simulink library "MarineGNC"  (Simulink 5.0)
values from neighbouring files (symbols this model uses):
  D = 6.533    [RRDcontainer.m]    (also in ExObsCtr.m = sqrt(g/L)*T*Dbis*Tinv)
  delta_max = 20    [RRDcontainer.m]
  G = Hmtrx(r_g)' * G_CG * Hmtrx(r_g)    [Gmtrx.m]    (also in ExLQR.m = -K; ExRRD1.m = [ 0 0.0000704  0; ExRRD2.m = [ 0 0.0000704  0)
  M = 1    [ExWindForce.m]    (also in ExRRD1.m = [ 0.01497    0.0003525     -0.0002205; ExRRD2.m = [ 0.01497    0.0003525     -0.0002205; ExObsCtr.m = T*Mbis*Tinv)
  pathlength = pathlength + sqrt( (xpath(j+1)-xpath(j))^2 + (ypath(j+1)-ypath(j))^2)    [order5.m]    (also in order3.m)
  table = table'    [order5.m]    (also in order3.m)
undefined symbols (not defined in the file or in its folder): Acc, feval, K_supply, rate_max, T_supply
libraries: MarineGNC x24, simulink x18
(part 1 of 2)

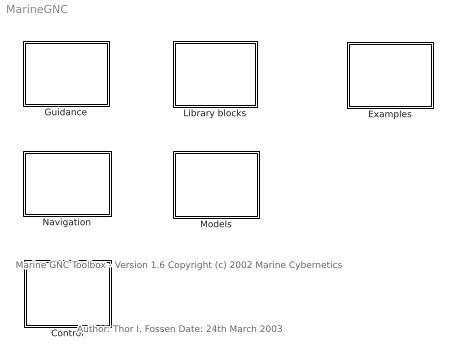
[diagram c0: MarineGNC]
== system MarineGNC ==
  note: Marine GNC Toolbox - Version 1.6 Copyright (c) 2002 Marine Cybernetics
  note: Author: Thor I. Fossen Date: 24th March 2003
  Control : Subsystem
  Examples : Subsystem
  Guidance : Subsystem
  Library blocks : Subsystem
  Models : Subsystem
  Navigation : Subsystem

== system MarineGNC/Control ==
  Ship control systems : Subsystem

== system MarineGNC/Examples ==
  Autopilot wave filter:   compass and yaw gyro : Subsystem
  Autopilot with wave filter: only compass measurement : Subsystem
  "Simulink interface for  m-file vessel models " : Subsystem
  Thruster configuration matrix for supply vessel : Subsystem
  Way-point guidance : Subsystem

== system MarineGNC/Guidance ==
  Reference model : Subsystem  mask(3rd-order reference model){v_max=1.0, zeta_d=1.0, w_d=0.1}
      mask prompts: v_max "Max. velocity:"; zeta_d "Relative damping ratio:"; w_d "Natural frequency:"
      mask help: 3rd-order reference model with velocity saturation.
  Way-point guidance block : Subsystem  mask(Guidance){x_vector=[-800 -500 -200 -50 -200 -250 200 500 500 300 0 -300 -600], y_vector=[100 1800 2000 1500 1000 100 1000 300 -250 -200 100 -600 -1000], method=5th order polynomial, drawmode=off, stop=on, mode=Acc, start=[100 0], final=[0 100], constraint=off}
      mask prompts: x_vector "X value"; y_vector "Y value"; method "Computation method for path generation"; drawmode "Draw an extra plot showing the path with waypoints"; stop "Stop simulation when last waypoint is reached"; mode "Use constraints on acceleration or velocity in the endpoints"; start "Constraints in first waypoint [x, y]. (Only applicable for cubic splines)"; final "Constraints in last waypoint [x, y]. (Only applicable for cubic splines)"; constraint "Use constraints on the derivatives (Only applicable for 5th order)"
      mask help: Way-Point Guidance Block Author: Jørgen Corneliussen Date: 20 November 2002 Creates a three times differentiable path between the waypoints provided. The user can choose between cubic splines and polinomial interpolation. NOTE: You have to supply the actual waypoints for the path generation.
      mask init:
      | if method == 1
      | 	[table, pathlength] = order3(x_vector,y_vector, drawmode, mode, start(1), final(1), start(2), final(2));
      | elseif method == 2
      | 	[table, pathlength] = order5(drawmode, constraint, x_vector, y_vector);
      | else
      | 	disp('Error in block initialization')
      | end

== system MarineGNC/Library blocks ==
  Angle conversion : Subsystem
  Axes transformations : Subsystem
  Equations of motion : Subsystem

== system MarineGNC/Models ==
  Actuators : Subsystem
  Vessels : Subsystem
  "Waves, wind and currents" : Subsystem

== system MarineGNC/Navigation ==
  Wave filters : Subsystem

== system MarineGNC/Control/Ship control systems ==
  Course autopilot : Subsystem  mask(Course Autopilot){T_nomoto=1, K_nomoto=1, Kp=1, Td=0, Ti=0}
      mask prompts: T_nomoto "Nomoto Time Constant: T"; K_nomoto "Nomoto gain: K"; Kp "Proportional Gain: Kp"; Td "Derivative Time: Td"; Ti "Integral Time: Ti"
      mask help: PID Autopilot with reference feedforward.
  DP controller : Subsystem  mask(Nonlinear DP Controller){Kp=diag([1 1 1]), Kd=diag([1 1 1]), Ki=diag([1 1 1])}
      mask prompts: Kp "Proportional Gain Matrix: Kp"; Kd "Derivative Gain Matrix: Kd"; Ki "Integral Gain Matrix: Ki"
      mask help: Nonlinear PID controller for Set-Point Reulation in Surge, Sway and Yaw

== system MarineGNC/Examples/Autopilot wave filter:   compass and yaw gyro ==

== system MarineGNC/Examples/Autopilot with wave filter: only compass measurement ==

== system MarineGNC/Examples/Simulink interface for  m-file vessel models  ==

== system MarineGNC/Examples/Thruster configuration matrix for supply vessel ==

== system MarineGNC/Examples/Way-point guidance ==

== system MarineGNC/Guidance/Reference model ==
  desired position : Inport
  "    " : TransferFcn  Denominator=[1 0]
  "       " : Saturate  UpperLimit=v_max  LowerLimit=-v_max
  "         " : TransferFcn  Denominator=[1 0]
  Sum2 : Sum  Inputs=|+-
  Sum5 : Sum  Inputs=|+-
  damping : Gain  Orientation=left  Gain=2*zeta_d*w_d
  low-pass filter : TransferFcn  Numerator=[w_d^3]  Denominator=[1 w_d]
  spring : Gain  Orientation=left  Gain=w_d*w_d
  "desired position " : Outport  InitialOutput=0
  desired velocity : Outport  Port=2  InitialOutput=0
  desired acceleration : Outport  Port=3  InitialOutput=0
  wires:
  damping/1 -> Sum5/2
  "         "/1 -> "       "/1
  "    "/1 -> "desired position "/1, spring/1
  spring/1 -> Sum2/2
  Sum2/1 -> Sum5/1
  low-pass filter/1 -> Sum2/1
  desired position/1 -> low-pass filter/1
  Sum5/1 -> "         "/1, desired acceleration/1
  "       "/1 -> damping/1, "    "/1, desired velocity/1

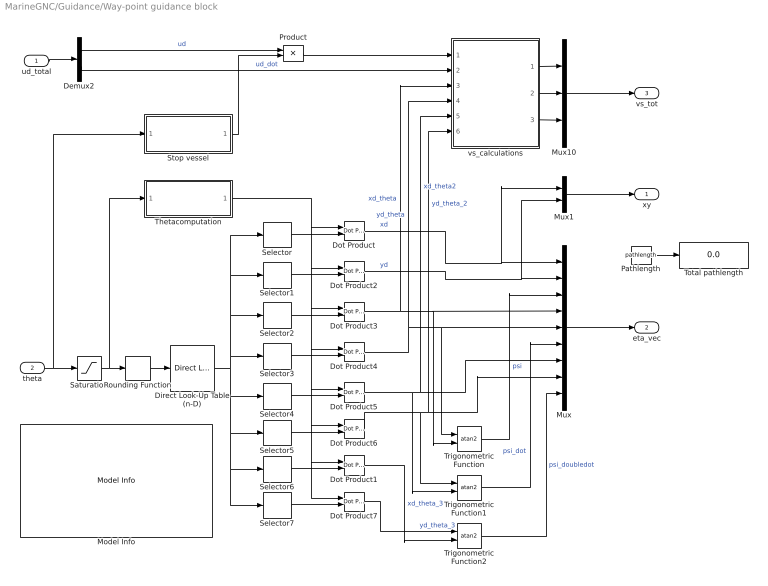
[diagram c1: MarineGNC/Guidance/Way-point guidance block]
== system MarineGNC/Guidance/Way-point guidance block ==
  ud_total : Inport  PortDimensions=2
  theta : Inport  Port=2
  Demux2 : Demux  Outputs=2
  Direct Look-Up Table (n-D) : simulink/Look-Up Tables/Direct Look-Up Table (n-D)  maskTabDims=2  explicitNumDims=1  outDims=Column  tabIsInput=off  mxTable=table  clipFlag=None
  Dot Product{,1..7} (8 alike) : simulink/Math Operations/Dot Product
  Model Info : simulink/Model-Wide Utilities/Model Info  InitialBlockCM=none  BlockCM=None  Frame=on  DisplayStringWithTags=|  HorizontalTextAlignment=Center  LeftAlignmentValue=0.5  SourceBlockDiagram=MarineGNC  TagMaxNumber=20
      | Guidance block.
      | Creates a three times differentiable path 
      | between the provided waypoints. The user 
      | can choose between cubic splines and a 
      | 5th order polynomial.
      | Author: Jørgen Corneliussen
      | Modified: %<ModifiedDate>
      | Version: %<ModelVersion>
  Mux : Mux  Inputs=9
  Mux1 : Mux  Inputs=2
  Mux10 : Mux  Inputs=3
  Pathlength : Constant  Value=pathlength
  Product : Product
  Rounding Function : Rounding
  Saturation : Saturate  UpperLimit=size(table,2) -0.001  LowerLimit=0
  Selector : Selector  Elements=[0*(size(table,1)/8)+1 :1*(size(table,1)/8)]  InputPortWidth=size(table,1)
  Selector1 : Selector  Elements=[1*(size(table,1)/8)+1 :2*(size(table,1)/8)]  InputPortWidth=size(table,1)
  Selector2 : Selector  Elements=[2*(size(table,1)/8)+1 :3*(size(table,1)/8)]  InputPortWidth=size(table,1)
  Selector3 : Selector  Elements=[3*(size(table,1)/8)+1 :4*(size(table,1)/8)]  InputPortWidth=size(table,1)
  Selector4 : Selector  Elements=[4*(size(table,1)/8)+1 :5*(size(table,1)/8)]  InputPortWidth=size(table,1)
  Selector5 : Selector  Elements=[5*(size(table,1)/8)+1 :6*(size(table,1)/8)]  InputPortWidth=size(table,1)
  Selector6 : Selector  Elements=[6*(size(table,1)/8)+1 :7*(size(table,1)/8)]  InputPortWidth=size(table,1)
  Selector7 : Selector  Elements=[7*(size(table,1)/8)+1 :8*(size(table,1)/8)]  InputPortWidth=size(table,1)
  Stop vessel : Subsystem
  Thetacomputation : Subsystem
  Total pathlength : Display
  Trigonometric Function : Trigonometry  Operator=atan2
  Trigonometric Function1 : Trigonometry  Operator=atan2
  Trigonometric Function2 : Trigonometry  Operator=atan2
  vs_calculations : Subsystem
  xy : Outport
  eta_vec : Outport  Port=2
  vs_tot : Outport  Port=3
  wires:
  theta/1 -> Saturation/1, Stop vessel/1(theta)
  ud_total/1 -> Demux2/1
  Thetacomputation/1(thetavector) -> Dot Product/1, Dot Product2/1, Dot Product4/1, Dot Product5/1, Dot Product6/1, Dot Product7/1, Dot Product1/1, Dot Product3/1
  Dot Product/1 -> Mux/1, Mux1/1  "xd"
  Dot Product2/1 -> Mux/2, Mux1/2  "yd"
  Mux/1 -> eta_vec/1
  Dot Product3/1 -> Trigonometric Function/2, Mux/4, vs_calculations/3(xd_theta)  "xd_theta"
  Dot Product4/1 -> Mux/5, Trigonometric Function/1, vs_calculations/4(yd_theta)  "yd_theta"
  Dot Product5/1 -> Trigonometric Function1/2, Mux/7, vs_calculations/5(xd_theta_2)  "xd_theta2"
  Dot Product6/1 -> Trigonometric Function1/1, Mux/8, vs_calculations/6(yd_theta_2)  "yd_theta_2"
  Dot Product1/1 -> Trigonometric Function2/2  "xd_theta_3"
  Dot Product7/1 -> Trigonometric Function2/1  "yd_theta_3"
  Trigonometric Function/1 -> Mux/3  "psi"
  Trigonometric Function1/1 -> Mux/6  "psi_dot"
  Trigonometric Function2/1 -> Mux/9  "psi_doubledot"
  Mux10/1 -> vs_tot/1
  vs_calculations/1(vs) -> Mux10/1
  vs_calculations/3(vs_t) -> Mux10/3
  vs_calculations/2(vs_theta) -> Mux10/2
  Saturation/1 -> Rounding Function/1, Thetacomputation/1(theta)
  Selector/1 -> Dot Product/2
  Selector1/1 -> Dot Product2/2
  Selector2/1 -> Dot Product3/2
  Selector3/1 -> Dot Product4/2
  Selector4/1 -> Dot Product5/2
  Selector5/1 -> Dot Product6/2
  Selector6/1 -> Dot Product1/2
  Selector7/1 -> Dot Product7/2
  Direct Look-Up Table (n-D)/1 -> Selector/1, Selector1/1, Selector2/1, Selector3/1, Selector4/1, Selector5/1, Selector7/1, Selector6/1
  Rounding Function/1 -> Direct Look-Up Table (n-D)/1
  Demux2/1 -> Product/1  "ud"
  Product/1 -> vs_calculations/1(ud)
  Stop vessel/1(stopsignal) -> Product/2
  Demux2/2 -> vs_calculations/2(ud_dot)  "ud_dot"
  Mux1/1 -> xy/1
  Pathlength/1 -> Total pathlength/1

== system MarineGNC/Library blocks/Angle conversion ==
  deg to [-180 180] : Subsystem
  rad to [-pi pi] : Subsystem

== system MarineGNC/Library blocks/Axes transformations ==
  6 DOF transformation : Subsystem
  Euler angles to rotation matrix : Subsystem
  Euler angles to attitude transformation matrix : Subsystem
  "Rotataion matrix in yaw " : Subsystem
  Transformation of generalized force : Subsystem
  Transposed rotation  matrix in yaw : Subsystem

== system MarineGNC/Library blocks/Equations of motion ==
  3 DOF Eqs. of motion : Subsystem
  3 to 6 DOF : Subsystem
  6 DOF Eqs. of motion : Subsystem
  6 to 3 DOF : Selector  Elements=[1 2 6]  InputPortWidth=6

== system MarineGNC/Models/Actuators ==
  note: Propellers
  note: Thruster configuration blocks
  note: Machines
  Column vector t1 : Subsystem
  Propeller : Subsystem  mask(Propeller){rpm_max=5*(180/pi)}
      mask prompts: rpm_max "Max RPM:"
  Steering machine : Subsystem
  T(alpha) : Subsystem

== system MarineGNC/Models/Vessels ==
  note: Nomoto models (1 DOF)
  note: Low-Speed Models (3 DOF)
  note: Low-Speed Models (6 DOF) 6 DOF interface for 3 DOF models
  note: Interface to m-file models
  3 to 6 DOF : MarineGNC/Library blocks/Equations of motion/3 to 6 DOF
  3 to 6 DOF1 : MarineGNC/Library blocks/Equations of motion/3 to 6 DOF
  6 to 3 DOF : Selector  Elements=[1 2 6]  InputPortWidth=6
  CyberShipII : Subsystem  LoadFcn=initCS2
  Mariner class cargo ship  (2nd -order) : Subsystem  mask(Container ship (2nd-order model)){rate_max=5*(pi/180), delta_max=20*(pi/180), K=0.185, T1=118, T2=7.8, T3=18.5}
      mask prompts: rate_max "Max rudder rate: rate_max (rad/s)"; delta_max "Max rudder angle: delta_max (rad)"; K "Gain constant: K (1/s)"; T1 "Time constant: T1 (s)"; T2 "Time constant: T2 (s)"; T3 "Time constant: T3 (s)"
  Semi-sub : Subsystem  InitFcn=load MDGmodels/rig  mask(Semi-submersiblel (6 DOF)){D=D, G=G, M=M}
      mask prompts: D "Linear damping matrix: D"; G "Spring matrix G:"; M "System inertia matrix: M"
      mask help: Semi-submersible low-speed model for DP. Inputs: tau = 6 DOF control input vector (generalized force) Outputs: eta = [x, y, z, phi, theta, psi]' nu = [u, v, w, p, q, r]'
  Supply vessel : Subsystem  mask(Supply Vessel (surge, sway and yaw)){D=[5.0242e4 0 0; 0 2.7229e5 -4.3933e6; 0 -4.3933e6 4.1894e8], Minv=inv( [5.3122e6 0 0; 0 8.2831e6 0; 0 0 3.7454e9] )}
      mask prompts: D "Linear damping matrix: D"; Minv "Inverse inertia matrix: Minv"
      mask help: DP model Inputs: tau = 3 DOF control input vector (generalized force) Outputs: eta = [x, y, psi]' nu = [u, v, r]'
  Supply vessel1 : MarineGNC/Models/Vessels/Supply vessel  D=[5.0242e4 0 0; 0 2.7229e5 -4.3933e6; 0 -4.3933e6 4.1894e8]  Minv=inv( [5.3122e6 0 0; 0 8.2831e6 0; 0 0 3.7454e9] )
  Tanker (1st-order) : Subsystem  mask(Tanker (Nomoto 1st.-order)){rate_max=5*(pi/180), delta_max=20*(pi/180), K=-0.019, T=-153.7}
      mask prompts: rate_max "Max rudder rate: rate_max (rad/s):"; delta_max "Max rudder angle: delta_max  (rad)"; K "Gain constant: K (1/s)"; T "Time constant: T (s)"
      mask help: Tanker: Nomoto 1st-order model Input: delta_c = rudder angle command (rad) Outputs: psi = yaw angle (rad) r = yaw rate (rad) delta = rudder angle from steering machine (rad)
  Tanker (2nd-order) : Subsystem  mask(Tanker (Nomoto 2nd-order model)){rate_max=5*(pi/180), delta_max=20*(pi/180), K=-0.019, T1=-124.1, T2=16.4, T3=46}
      mask prompts: rate_max "Max rudder rate: rate_max (rad/s)"; delta_max "Max rudder angle: delta_max (rad)"; K "Gain constant: K (1/s)"; T1 "Time constant: T1 (s)"; T2 "Time constant: T2 (s)"; T3 "Time constant: T3 (s)"
      mask help: Tanker: Nomoto 2nd-order model Input: delta_c = rudder angle command (rad) Outputs: psi = yaw angle (rad) r = yaw rate (rad) delta = rudder angle from steering machine (rad)
  m-file interface : Subsystem  mask(m-file vessel model interface){vessmodel=, dimu_model=, dimx_model=}
      mask prompts: vessmodel "m-file vessel model"; dimu_model "dim u"; dimx_model "dim x"
      mask help: Simulink interface to the GNC toolbox m-file vessel models, type: >help vesselmodels in the Matlab command window. A Simulink demo file is found under examples (demomf.mdl). Inputs/outputs: u = control input vector of dimension dimu xo = initial state vector of dimension dimx x = state vector of dimension dimu
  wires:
  Supply vessel1/1 -> 3 to 6 DOF/1
  Supply vessel1/2 -> 3 to 6 DOF1/1
  6 to 3 DOF/1 -> Supply vessel1/1

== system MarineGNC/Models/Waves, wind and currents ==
  Linear 2nd-order  wave spectrum : Subsystem  mask{sigma=1, w_0=1, lambda=0.1}
      mask prompts: sigma "Wave spectrum gain: sigma  (m)"; w_0 "Wave spectrum peak frequency: w_0  (rad/s)"; lambda "Rrelative damping ratio: lambda"
      mask init:
      | w = 0.01:0.1:3*w_0;

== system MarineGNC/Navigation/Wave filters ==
  Passive autopilot wave filter 1 : Subsystem  mask(wave spectrum damping ratio){lambda=0.1, w_o=1.2, K4=0.1, K5=0.01, w_c=1.3, T=100, K=1, T_b=100}
      mask prompts: lambda "Relative damping ratio of wave spectrum: lambda"; w_o "Peak frequency of wave spectrum: w_o (rad/s)"; K4 "Yaw rate observer gain: K4"; K5 "Bias observer gain: K5"; w_c "Filter cut-off frequency: w_c (rad/s)"; T "Nomoto time constant: T (s)"; K "Nomoto gain: K (1/s)"; T_b "Rudder bias time constant: T_b (s)"
  Passive autopilot wave filter 2 : Subsystem  mask(wave spectrum damping ratio){lambda=0.1, w_o=1.2, K4=0.1, zeta_n=0.01, w_c=2, T_b=100}
      mask prompts: lambda "Relative damping ratio of wave spectrum: lambda"; w_o "Peak frequency of wave spectrum: w_o (rad/s)"; K4 "Bias observer gain: K4"; zeta_n "Relative damping ratio in gyro notch filter: zeta_n"; w_c "Filter cut-off frequency: w_c (rad/s)"; T_b "Bias time constant: T_b (s)"

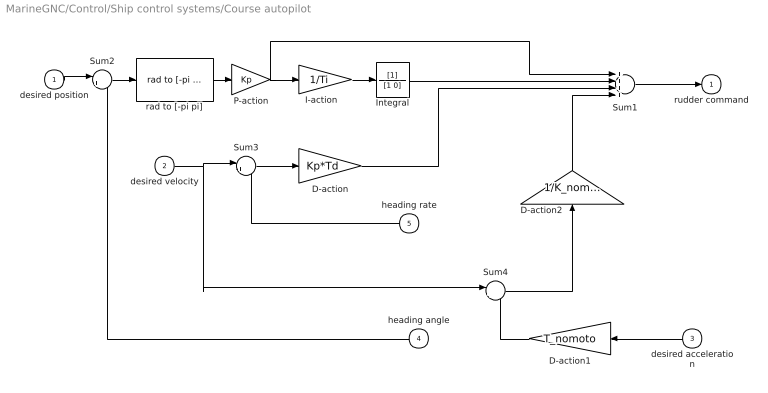
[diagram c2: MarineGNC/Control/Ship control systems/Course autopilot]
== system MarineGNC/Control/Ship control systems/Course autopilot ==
  desired position : Inport
  desired velocity : Inport  Port=2
  desired acceleration : Inport  Orientation=left  Port=3
  heading angle : Inport  Orientation=left  Port=4
  heading rate : Inport  Orientation=left  Port=5
  D-action : Gain  Gain=Kp*Td
  D-action1 : Gain  Orientation=left  Gain=T_nomoto
  D-action2 : Gain  Orientation=up  Gain=1/K_nomoto
  "I-action   " : Gain  Gain=1/Ti
  Integral : TransferFcn  Denominator=[1 0]
  P-action : Gain  Gain=Kp
  Sum1 : Sum  Inputs=++++
  Sum2 : Sum  Inputs=|+-
  Sum3 : Sum  Inputs=|+-
  Sum4 : Sum  Inputs=|++
  rad to [-pi pi] : MarineGNC/Library blocks/Angle conversion/rad to [-pi pi]  SimViewingDevice=off  DataTypeOverride=UseLocalSettings  MinMaxOverflowLogging=UseLocalSettings
  rudder command : Outport  InitialOutput=0
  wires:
  P-action/1 -> Sum1/1, "I-action   "/1
  "I-action   "/1 -> Integral/1
  D-action/1 -> Sum1/3
  Sum1/1 -> rudder command/1
  Integral/1 -> Sum1/2
  Sum3/1 -> D-action/1
  heading angle/1 -> Sum2/2
  desired acceleration/1 -> D-action1/1
  heading rate/1 -> Sum3/2
  desired velocity/1 -> Sum3/1, Sum4/1
  D-action1/1 -> Sum4/2
  Sum4/1 -> D-action2/1
  D-action2/1 -> Sum1/4
  Sum2/1 -> rad to [-pi pi]/1
  rad to [-pi pi]/1 -> P-action/1
  desired position/1 -> Sum2/1

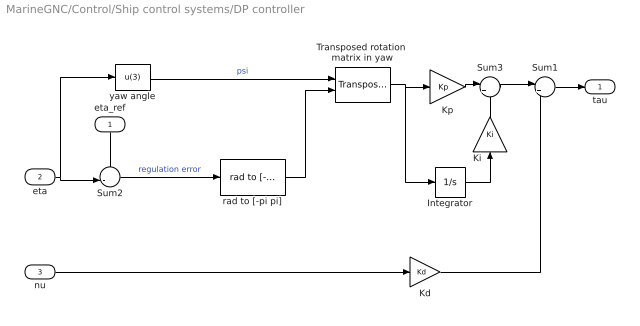
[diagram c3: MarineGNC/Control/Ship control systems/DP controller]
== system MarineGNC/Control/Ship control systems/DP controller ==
  eta_ref : Inport  Orientation=down
  eta : Inport  Port=2
  nu : Inport  Port=3
  Integrator : Integrator
  Kd : Gain  Gain=Kd  Multiplication=Matrix(K*u)
  Ki : Gain  Orientation=up  Gain=Ki  Multiplication=Matrix(K*u)
  Kp : Gain  Gain=Kp  Multiplication=Matrix(K*u)
  Sum1 : Sum  Inputs=|+-
  Sum2 : Sum  Inputs=+-|
  Sum3 : Sum  Inputs=|++
  Transposed rotation  matrix in yaw : MarineGNC/Library blocks/Axes transformations/Transposed rotation  matrix in yaw
  rad to [-pi pi] : MarineGNC/Library blocks/Angle conversion/rad to [-pi pi]  SimViewingDevice=off  DataTypeOverride=UseLocalSettings  MinMaxOverflowLogging=UseLocalSettings
  yaw angle : Fcn  Expr=u(3)
  tau : Outport  InitialOutput=0
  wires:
  Transposed rotation  matrix in yaw/1 -> Integrator/1, Kp/1
  Ki/1 -> Sum3/2
  Sum3/1 -> Sum1/1
  Kp/1 -> Sum3/1
  Integrator/1 -> Ki/1
  Kd/1 -> Sum1/2
  nu/1 -> Kd/1
  yaw angle/1 -> Transposed rotation  matrix in yaw/1  "psi"
  eta/1 -> yaw angle/1, Sum2/2
  Sum1/1 -> tau/1
  eta_ref/1 -> Sum2/1
  Sum2/1 -> rad to [-pi pi]/1  "regulation error"
  rad to [-pi pi]/1 -> Transposed rotation  matrix in yaw/2

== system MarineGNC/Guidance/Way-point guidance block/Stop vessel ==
  theta : Inport
  If endpoint1 : If  IfExpression=u1 > size(table,2)
  Merge : Merge
  Model Info : simulink/Model-Wide Utilities/Model Info  InitialBlockCM=None  BlockCM=None  Frame=on  DisplayStringWithTags=|  HorizontalTextAlignment=Center  LeftAlignmentValue=0.5  SourceBlockDiagram=demowpt  TagMaxNumber=20
      | Stop vessel
      | 
      | This subsystem performs an action when
      | the vessel reaches the last waypoint. The 
      | simultation is either stopped, or the desired 
      | speed is set to zero.
      | 
      | Author: Jørgen Corneliussen
      | Modified: %<ModifiedDate>
      | Version: %<ModelVersion>
  Reached endpoint : Subsystem  TreatAsAtomicUnit=on
  Still travelling : Subsystem  TreatAsAtomicUnit=on
  stopsignal : Outport
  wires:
  Still travelling/1(one) -> Merge/2
  theta/1 -> If endpoint1/1
  If endpoint1/1 -> Reached endpoint/Action
  Reached endpoint/1(zero) -> Merge/1
  Merge/1 -> stopsignal/1
  If endpoint1/2 -> Still travelling/Action

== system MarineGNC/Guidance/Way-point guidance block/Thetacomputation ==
  theta : Inport
  5th order algorithm : Subsystem  TreatAsAtomicUnit=on
  Constant1 : Constant  Value=method
  Cubic splines : Subsystem  TreatAsAtomicUnit=on
  If endpoint1 : If  IfExpression=u1 == 1
  Model Info : simulink/Model-Wide Utilities/Model Info  InitialBlockCM=None  BlockCM=None  Frame=on  DisplayStringWithTags=|  HorizontalTextAlignment=Center  LeftAlignmentValue=0.5  SourceBlockDiagram=demowpt  TagMaxNumber=20
      | Thetacomputation
      | This subsystem returns a vector containing 
      | different orders of theta.
      | 
      | If cubic splines is used, the system returns:
      | [th^3 th^2 th 1]
      | 
      | If the 5th order polynomial is used, it returns:
      | [th^5 th^4 th^3 th^2 th 1]
      | 
      | Author: Jørgen Corneliussen
      | Modified: %<ModifiedDate>
      | Version: %<ModelVersion>
  Multiport Switch : MultiPortSwitch  Inputs=2
  Selector : Selector  Elements=[1:size(table,1)/8]  InputPortWidth=6
  thetavector : Outport
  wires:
  If endpoint1/1 -> Cubic splines/Action  "cubic"
  If endpoint1/2 -> 5th order algorithm/Action
  Constant1/1 -> If endpoint1/1, Multiport Switch/1
  theta/1 -> 5th order algorithm/1(theta), Cubic splines/1(theta)
  5th order algorithm/1(theta_vector) -> Multiport Switch/3
  Selector/1 -> thetavector/1
  Cubic splines/1(theta_vector) -> Multiport Switch/2
  Multiport Switch/1 -> Selector/1

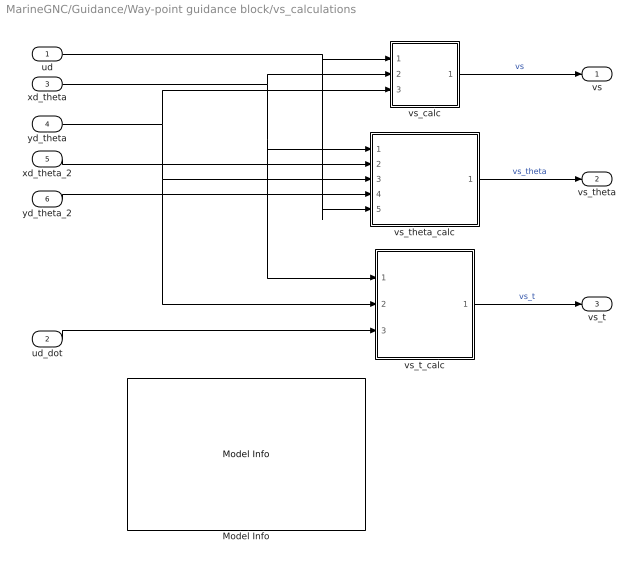
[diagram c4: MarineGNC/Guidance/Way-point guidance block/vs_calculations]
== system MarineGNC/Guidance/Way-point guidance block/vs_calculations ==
  ud : Inport
  ud_dot : Inport  Port=2
  xd_theta : Inport  Port=3
  yd_theta : Inport  Port=4
  xd_theta_2 : Inport  Port=5
  yd_theta_2 : Inport  Port=6
  Model Info : simulink/Model-Wide Utilities/Model Info  InitialBlockCM=None  BlockCM=None  Frame=on  DisplayStringWithTags=|  HorizontalTextAlignment=Center  LeftAlignmentValue=0.5  SourceBlockDiagram=demowpt  TagMaxNumber=20
      | vs_calculations
      | 
      | This subsystem returns a vector containing 
      | the  speed assignment along the path.
      | The vector contains the desired speed, and 
      | the derivative of the desired speed with regards
      |  to theta and with regards to time.
      | 
      | Author: Jørgen Corneliussen
      | Modified: %<ModifiedDate>
      | Version: %<ModelVersion>
  vs_calc : Subsystem
  vs_t_calc : Subsystem
  vs_theta_calc : Subsystem
  vs : Outport
  vs_theta : Outport  Port=2
  vs_t : Outport  Port=3
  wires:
  vs_calc/1(vs) -> vs/1  "vs"
  vs_theta_calc/1(vs_theta) -> vs_theta/1  "vs_theta"
  vs_t_calc/1(vs_t) -> vs_t/1  "vs_t"
  ud/1 -> vs_calc/1(ud), vs_theta_calc/5(ud)
  ud_dot/1 -> vs_t_calc/3(ud_dot)
  xd_theta/1 -> vs_calc/2(xd_theta), vs_theta_calc/1(xd_theta), vs_t_calc/1(xd_theta)
  yd_theta/1 -> vs_calc/3(yd_theta), vs_theta_calc/3(yd_theta), vs_t_calc/2(yd_theta)
  xd_theta_2/1 -> vs_theta_calc/2(xd_theta_2)
  yd_theta_2/1 -> vs_theta_calc/4(yd_theta_2)

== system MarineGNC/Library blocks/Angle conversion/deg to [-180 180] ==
  y (deg) : Inport
  Constant : Constant  Value=180
  Constant1 : Constant  Value=-180
  Data Type Conversion : DataTypeConversion  DataType=double
  "Data Type Conversion  " : DataTypeConversion  DataType=double
  Relational Operator : RelationalOperator  Operator=>
  Relational Operator1 : RelationalOperator  Operator=<
  Sum2 : Sum  Inputs=+++
  twopi : Gain  Gain=-2*180
  "twopi  " : Gain  Gain=2*180
  -180<y180 : Outport  InitialOutput=0
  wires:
  Constant/1 -> Relational Operator/2
  Relational Operator/1 -> Data Type Conversion/1
  Constant1/1 -> Relational Operator1/2
  Relational Operator1/1 -> "Data Type Conversion  "/1
  twopi/1 -> Sum2/1
  "twopi  "/1 -> Sum2/3
  Sum2/1 -> -180<y180/1  "add"
  y (deg)/1 -> Sum2/2, Relational Operator1/1, Relational Operator/1
  Data Type Conversion/1 -> twopi/1
  "Data Type Conversion  "/1 -> "twopi  "/1

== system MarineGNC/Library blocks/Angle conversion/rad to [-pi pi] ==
  y (rad) : Inport
  Constant : Constant  Value=pi
  "Constant " : Constant  Value=-pi
  Data Type Conversion : DataTypeConversion  DataType=double
  Data Type Conversion1 : DataTypeConversion  DataType=double
  Relational Operator : RelationalOperator  Operator=>
  Relational Operator1 : RelationalOperator  Operator=<
  Sum2 : Sum  Inputs=+++
  two pi : Gain  Gain=-2*pi
  "two pi  " : Gain  Gain=2*pi
  -pi<y<pi : Outport  InitialOutput=0
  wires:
  Constant/1 -> Relational Operator/2
  Relational Operator/1 -> Data Type Conversion/1
  "Constant "/1 -> Relational Operator1/2
  Relational Operator1/1 -> Data Type Conversion1/1
  two pi/1 -> Sum2/1
  "two pi  "/1 -> Sum2/3
  Sum2/1 -> -pi<y<pi/1  "add"
  y (rad)/1 -> Sum2/2, Relational Operator1/1, Relational Operator/1
  Data Type Conversion/1 -> two pi/1
  Data Type Conversion1/1 -> "two pi  "/1

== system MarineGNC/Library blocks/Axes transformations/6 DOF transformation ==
  note: Theta
  note: v
  note: omega
  eta : Inport
  nu : Inport  Port=2
  Euler angles to rotation matrix : MarineGNC/Library blocks/Axes transformations/Euler angles to rotation matrix
  Euler angles to attitude transformation matrix : MarineGNC/Library blocks/Axes transformations/Euler angles to attitude transformation matrix
  Mux : Mux  Inputs=2
  Product : Product  Inputs=**  Multiplication=Matrix(*)  ShowAdditionalParam=on
  Product1 : Product  Inputs=**  Multiplication=Matrix(*)  ShowAdditionalParam=on
  Selector : Selector  Elements=[4 5 6]  InputPortWidth=6
  Selector1 : Selector  Elements=[1 2 3]  InputPortWidth=6
  Selector2 : Selector  Elements=[4 5 6]  InputPortWidth=6
  J(eta)*nu : Outport
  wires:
  Selector/1 -> Euler angles to rotation matrix/1, Euler angles to attitude transformation matrix/1
  eta/1 -> Selector/1
  Euler angles to rotation matrix/1 -> Product/1
  nu/1 -> Selector1/1, Selector2/1
  Selector1/1 -> Product/2
  Selector2/1 -> Product1/2
  Euler angles to attitude transformation matrix/1 -> Product1/1
  Product/1 -> Mux/1
  Mux/1 -> J(eta)*nu/1
  Product1/1 -> Mux/2

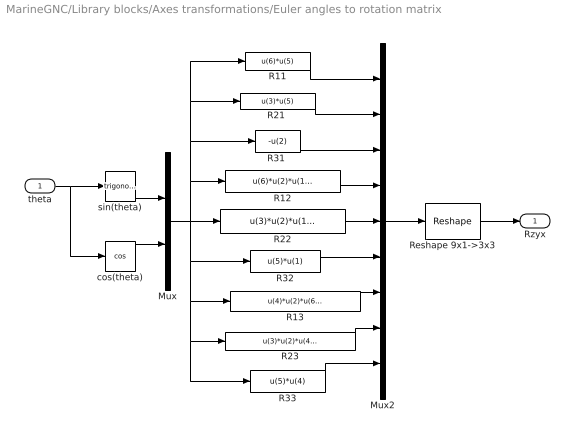
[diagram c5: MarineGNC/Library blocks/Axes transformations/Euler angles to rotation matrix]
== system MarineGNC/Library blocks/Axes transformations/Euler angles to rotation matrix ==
  theta : Inport
  Mux : Mux  Inputs=2
  Mux2 : Mux  Inputs=9
  R11 : Fcn  Expr=u(6)*u(5)
  R12 : Fcn  Expr=u(6)*u(2)*u(1)-u(3)*u(4)
  R13 : Fcn  Expr=u(4)*u(2)*u(6)+u(3)*u(1)
  "R21 " : Fcn  Expr=u(3)*u(5)
  R22 : Fcn  Expr=u(3)*u(2)*u(1)+u(6)*u(4)
  R23 : Fcn  Expr=u(3)*u(2)*u(4)-u(6)*u(1)
  "R31 " : Fcn  Expr=-u(2)
  R32 : Fcn  Expr=u(5)*u(1)
  R33 : Fcn  Expr=u(5)*u(4)
  Reshape 9x1->3x3 : simulink/Math Operations/Reshape  OutputDimensionality=Customize  OutputDimensions=[3,3]
  cos(theta) : Trigonometry  Operator=cos
  sin(theta) : Trigonometry
  Rzyx : Outport  InitialOutput=0
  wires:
  R11/1 -> Mux2/1
  Mux2/1 -> Reshape 9x1->3x3/1
  Reshape 9x1->3x3/1 -> Rzyx/1
  sin(theta)/1 -> Mux/1
  cos(theta)/1 -> Mux/2
  theta/1 -> sin(theta)/1, cos(theta)/1
  Mux/1 -> R32/1, R13/1, R33/1, R23/1, R22/1, "R31 "/1, R11/1, "R21 "/1, R12/1
  R23/1 -> Mux2/8
  R13/1 -> Mux2/7
  R22/1 -> Mux2/5
  R12/1 -> Mux2/4
  "R31 "/1 -> Mux2/3
  "R21 "/1 -> Mux2/2
  R32/1 -> Mux2/6
  R33/1 -> Mux2/9

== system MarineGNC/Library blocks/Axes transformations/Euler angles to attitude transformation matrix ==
  theta : Inport
  Constant : Constant
  "Constant " : Constant  Value=0
  Mux2 : Mux  Inputs=9
  Reshape 9x1->3x3 : simulink/Math Operations/Reshape  OutputDimensionality=Customize  OutputDimensions=[3,3]
  "T21 " : Fcn  Expr=sin(u(1))*tan(u(2))
  T22 : Fcn  Expr=cos(u(1))
  T23 : Fcn  Expr=sin(u(1))/cos(u(2))
  "T31 " : Fcn  Expr=cos(u(1))*tan(u(2))
  T32 : Fcn  Expr=-sin(u(1))
  T33 : Fcn  Expr=cos(u(1))/cos(u(2))
  T : Outport  InitialOutput=0
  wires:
  Constant/1 -> Mux2/1
  Mux2/1 -> Reshape 9x1->3x3/1
  Reshape 9x1->3x3/1 -> T/1
  theta/1 -> T23/1, T33/1, T32/1, "T31 "/1, T22/1, "T21 "/1
  T23/1 -> Mux2/6
  T22/1 -> Mux2/5
  T33/1 -> Mux2/9
  "Constant "/1 -> Mux2/2, Mux2/3
  "T21 "/1 -> Mux2/4
  "T31 "/1 -> Mux2/7
  T32/1 -> Mux2/8

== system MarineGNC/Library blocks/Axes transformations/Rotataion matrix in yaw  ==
  psi : Inport
  nu : Inport  Port=2
  Fcn : Fcn  Expr=cos(u(1))*u(2)-sin(u(1))*u(3)
  Fcn1 : Fcn  Expr=sin(u(1))*u(2)+cos(u(1))*u(3)
  Fcn2 : Fcn  Expr=u(4)
  Mux : Mux  Inputs=2
  Mux1 : Mux  Inputs=3
  R*nu : Outport
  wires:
  Mux/1 -> Fcn2/1, Fcn1/1, Fcn/1
  Fcn/1 -> Mux1/1  "x_dot"
  Fcn1/1 -> Mux1/2  "y_dot"
  Fcn2/1 -> Mux1/3  "psi_dot"
  Mux1/1 -> R*nu/1  "eta_dot"
  psi/1 -> Mux/1
  nu/1 -> Mux/2

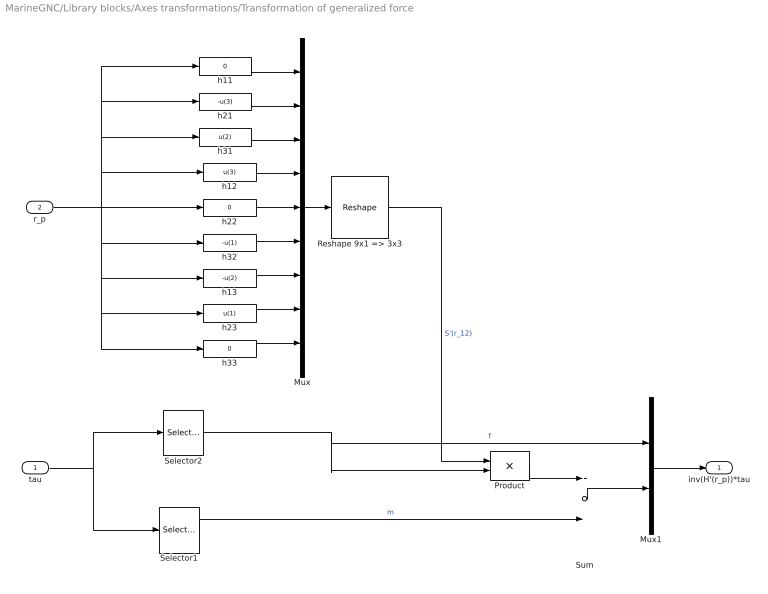
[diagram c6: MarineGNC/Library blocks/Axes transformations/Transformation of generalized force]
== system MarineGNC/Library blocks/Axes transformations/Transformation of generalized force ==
  tau : Inport
  r_p : Inport  Port=2
  Mux : Mux  Inputs=9
  Mux1 : Mux  Inputs=2
  Product : Product  Multiplication=Matrix(*)
  Reshape 9x1 => 3x3 : simulink/Math Operations/Reshape  OutputDimensionality=Customize  OutputDimensions=[3,3]
  Selector1 : Selector  Elements=[4 5 6]  InputPortWidth=6
  Selector2 : Selector  Elements=[1 2 3]  InputPortWidth=6
  Sum : Sum
  h11 : Fcn  Expr=0
  h12 : Fcn  Expr=u(3)
  h13 : Fcn  Expr=-u(2)
  h21 : Fcn  Expr=-u(3)
  h22 : Fcn  Expr=0
  h23 : Fcn  Expr=u(1)
  h31 : Fcn  Expr=u(2)
  h32 : Fcn  Expr=-u(1)
  h33 : Fcn  Expr=0
  inv(H'(r_p))*tau : Outport
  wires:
  tau/1 -> Selector1/1, Selector2/1
  Selector1/1 -> Sum/2  "m"
  Mux/1 -> Reshape 9x1 => 3x3/1
  Reshape 9x1 => 3x3/1 -> Product/1  "S'(r_12)"
  h11/1 -> Mux/1
  h21/1 -> Mux/2
  h31/1 -> Mux/3
  h12/1 -> Mux/4
  h22/1 -> Mux/5
  h32/1 -> Mux/6
  h13/1 -> Mux/7
  h23/1 -> Mux/8
  h33/1 -> Mux/9
  r_p/1 -> h11/1, h21/1, h31/1, h12/1, h22/1, h32/1, h13/1, h23/1, h33/1
  Mux1/1 -> inv(H'(r_p))*tau/1
  Selector2/1 -> Mux1/1, Product/2  "f"
  Sum/1 -> Mux1/2
  Product/1 -> Sum/1

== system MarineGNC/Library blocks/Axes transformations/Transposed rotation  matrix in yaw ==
  psi : Inport
  nu : Inport  Port=2
  Mux : Mux  Inputs=2
  Mux1 : Mux  Inputs=3
  Row1 : Fcn  Expr=cos(u(1))*u(2)+sin(u(1))*u(3)
  Row2 : Fcn  Expr=-sin(u(1))*u(2)+cos(u(1))*u(3)
  Row3 : Fcn  Expr=u(4)
  Out1 : Outport
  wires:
  nu/1 -> Mux/2
  psi/1 -> Mux/1
  Mux1/1 -> Out1/1
  Row3/1 -> Mux1/3
  Row2/1 -> Mux1/2
  Row1/1 -> Mux1/1
  Mux/1 -> Row1/1, Row2/1, Row3/1

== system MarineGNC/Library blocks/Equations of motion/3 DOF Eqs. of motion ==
  M : Inport
  tau : Inport  Port=2
  Integrator1 : Integrator
  Integrator2 : Integrator
  Product : Product  Inputs=/*  Multiplication=Matrix(*)
  "Rotataion matrix in yaw " : MarineGNC/Library blocks/Axes transformations/Rotataion matrix in yaw 
  Selector2 : Selector  Elements=[3]  InputPortWidth=3
  eta : Outport
  nu : Outport  Port=2
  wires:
  M/1 -> Product/1
  tau/1 -> Product/2
  Product/1 -> Integrator1/1  "d(nu)/dt"
  Integrator1/1 -> "Rotataion matrix in yaw "/2, nu/1  "nu"
  "Rotataion matrix in yaw "/1 -> Integrator2/1  "d(eta)/dt"
  Integrator2/1 -> Selector2/1, eta/1  "eta"
  Selector2/1 -> "Rotataion matrix in yaw "/1  "psi"

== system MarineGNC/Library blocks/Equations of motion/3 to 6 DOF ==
  In1 : Inport
  Constant : Constant  Value=0
  Mux1 : Mux  Inputs=2
  Selector : Selector  Elements="[1 2  4 4 4 3]"  InputPortWidth=4
  Out1 : Outport
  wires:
  Selector/1 -> Out1/1
  In1/1 -> Mux1/1
  Constant/1 -> Mux1/2
  Mux1/1 -> Selector/1

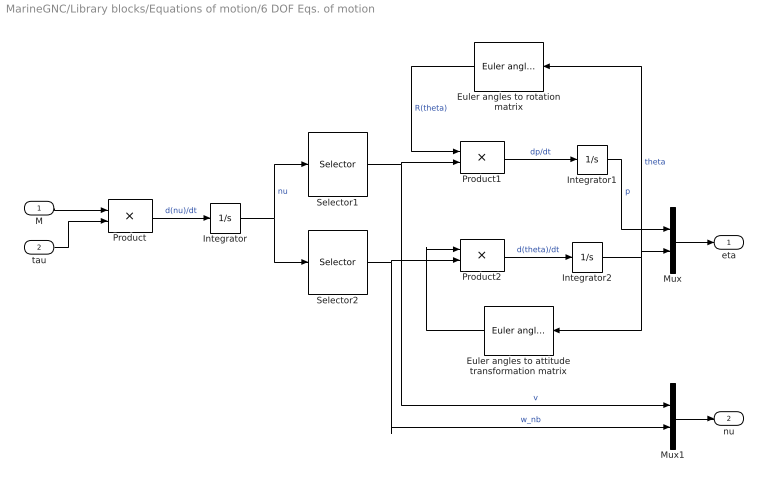
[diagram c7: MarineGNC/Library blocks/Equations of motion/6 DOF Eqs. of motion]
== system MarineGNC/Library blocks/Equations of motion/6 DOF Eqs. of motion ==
  M : Inport
  tau : Inport  Port=2
  Euler angles to rotation matrix : MarineGNC/Library blocks/Axes transformations/Euler angles to rotation matrix  Orientation=left
  Euler angles to attitude transformation matrix : MarineGNC/Library blocks/Axes transformations/Euler angles to attitude transformation matrix  Orientation=left
  Integrator : Integrator
  Integrator1 : Integrator
  Integrator2 : Integrator
  Mux : Mux  Inputs=2
  Mux1 : Mux  Inputs=2
  Product : Product  Inputs=/*  Multiplication=Matrix(*)
  Product1 : Product  Inputs=**  Multiplication=Matrix(*)
  Product2 : Product  Inputs=**  Multiplication=Matrix(*)
  Selector1 : Selector  Elements=[1 2 3]  InputPortWidth=6
  Selector2 : Selector  Elements=[4 5 6]  InputPortWidth=6
  eta : Outport
  nu : Outport  Port=2
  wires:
  M/1 -> Product/1
  tau/1 -> Product/2
  Product/1 -> Integrator/1  "d(nu)/dt"
  Integrator/1 -> Selector1/1, Selector2/1  "nu"
  Selector1/1 -> Product1/2, Mux1/1  "v"
  Selector2/1 -> Mux1/2, Product2/2  "w_nb"
  Product1/1 -> Integrator1/1  "dp/dt"
  Euler angles to rotation matrix/1 -> Product1/1  "R(theta)"
  Product2/1 -> Integrator2/1  "d(theta)/dt"
  Integrator2/1 -> Mux/2, Euler angles to rotation matrix/1, Euler angles to attitude transformation matrix/1  "theta"
  Integrator1/1 -> Mux/1  "p"
  Mux/1 -> eta/1
  Mux1/1 -> nu/1
  Euler angles to attitude transformation matrix/1 -> Product2/1

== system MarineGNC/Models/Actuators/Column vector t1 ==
  alpha : Inport
  lx : Inport  Port=2
  ly : Inport  Port=3
  "  " : Trigonometry  Operator=cos
  "   " : Trigonometry
  "    " : Product
  "       " : Product
  Sum : Sum  Inputs=|-+
  Thruster column vector : simulink/Math Operations/Matrix Concatenation  numInports=3  catMethod=Vertical
  t : Outport
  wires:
  "  "/1 -> Thruster column vector/1, "       "/1
  "   "/1 -> Thruster column vector/2, "    "/1
  alpha/1 -> "  "/1, "   "/1
  Thruster column vector/1 -> t/1
  "       "/1 -> Sum/1
  lx/1 -> "    "/2
  "    "/1 -> Sum/2
  Sum/1 -> Thruster column vector/3
  ly/1 -> "       "/2

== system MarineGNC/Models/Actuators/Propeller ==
  RPM command : Inport
  Propeller dynamics : Subsystem
  RPM : Outport
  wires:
  RPM command/1 -> Propeller dynamics/1(RPM_c)
  Propeller dynamics/1(RPM) -> RPM/1

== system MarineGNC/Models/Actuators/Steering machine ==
  delta_c : Inport
  Integrator : Integrator
  Sum : Sum  Inputs=|+-
  rudder angle saturation : Saturate  UpperLimit=delta_max  LowerLimit=-delta_max
  rudder rate saturation : Saturate  UpperLimit=rate_max  LowerLimit=-rate_max
  delta : Outport
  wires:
  rudder rate saturation/1 -> Integrator/1
  Sum/1 -> rudder rate saturation/1
  rudder angle saturation/1 -> Sum/1
  Integrator/1 -> delta/1, Sum/2
  delta_c/1 -> rudder angle saturation/1

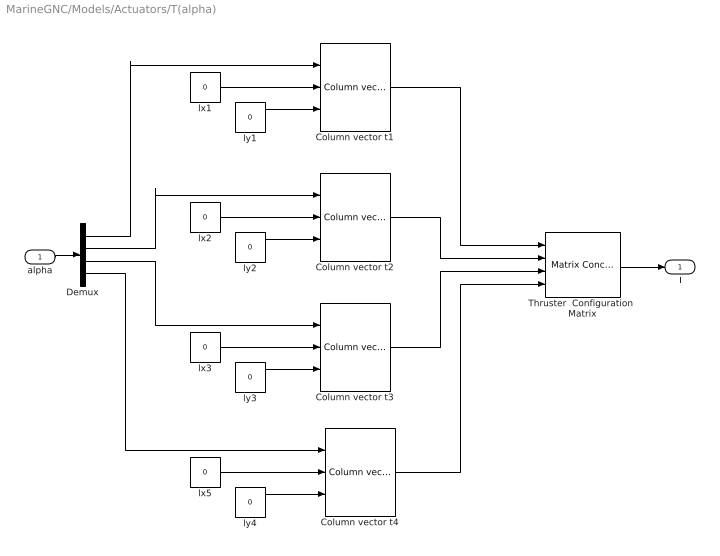
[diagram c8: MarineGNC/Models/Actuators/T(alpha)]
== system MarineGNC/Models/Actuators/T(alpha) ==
  alpha : Inport
  Column vector t{1..4} (4 alike) : MarineGNC/Models/Actuators/Column vector t1  SimViewingDevice=off  DataTypeOverride=UseLocalSettings  MinMaxOverflowLogging=UseLocalSettings
  Demux : Demux
  Thruster  Configuration  Matrix : simulink/Math Operations/Matrix Concatenation  numInports=4  catMethod=Horizontal
  lx{1..3,5} (4 alike) : Constant  Value=0
  ly{1..4} (4 alike) : Constant  Value=0
  T : Outport
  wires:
  Column vector t1/1 -> Thruster  Configuration  Matrix/1
  Column vector t2/1 -> Thruster  Configuration  Matrix/2
  Column vector t3/1 -> Thruster  Configuration  Matrix/3
  Column vector t4/1 -> Thruster  Configuration  Matrix/4
  Demux/1 -> Column vector t1/1
  Demux/2 -> Column vector t2/1
  Demux/3 -> Column vector t3/1
  Demux/4 -> Column vector t4/1
  alpha/1 -> Demux/1
  Thruster  Configuration  Matrix/1 -> T/1
  lx1/1 -> Column vector t1/2
  ly1/1 -> Column vector t1/3
  lx2/1 -> Column vector t2/2
  ly2/1 -> Column vector t2/3
  lx3/1 -> Column vector t3/2
  ly3/1 -> Column vector t3/3
  lx5/1 -> Column vector t4/2
  ly4/1 -> Column vector t4/3

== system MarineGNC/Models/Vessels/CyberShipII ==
  note: nu
  note: nu_dot
  note: etadot
  tau : Inport
  D : Gain  Orientation=left  Gain=D  Multiplication=Matrix(K*u)
  Integrator1 : Integrator
  Integrator2 : Integrator
  "Rotataion matrix in yaw " : Subsystem
  Sum3 : Sum  Inputs=+-
  inv(M) : Gain  Gain=inv(M)  Multiplication=Matrix(K*u)
  psi : Selector  Orientation=left  Elements=[3]  InputPortWidth=3
  saturation : Subsystem
  eta : Outport
  nu : Outport  Port=2
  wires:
  tau/1 -> saturation/1(tau)
  Integrator2/1 -> "Rotataion matrix in yaw "/2(nu), nu/1, D/1
  D/1 -> Sum3/2
  Sum3/1 -> inv(M)/1
  inv(M)/1 -> Integrator2/1
  "Rotataion matrix in yaw "/1(R*nu) -> Integrator1/1
  Integrator1/1 -> eta/1, psi/1
  psi/1 -> "Rotataion matrix in yaw "/1(psi)
  saturation/1(sat_tau) -> Sum3/1

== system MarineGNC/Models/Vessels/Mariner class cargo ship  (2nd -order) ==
  rudder command : Inport
  Ship model : Subsystem
  Steering machine : MarineGNC/Models/Actuators/Steering machine
  heading angle : Outport
  heading rate : Outport  Port=2
  rudder angle : Outport  Port=3
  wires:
  Ship model/2(heading rate) -> heading rate/1
  Ship model/1(heading angle) -> heading angle/1
  rudder command/1 -> Steering machine/1
  Steering machine/1 -> rudder angle/1, Ship model/1(rudder angle)

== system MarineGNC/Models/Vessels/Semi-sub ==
  tau : Inport
  6 DOF Eqs. of motion : MarineGNC/Library blocks/Equations of motion/6 DOF Eqs. of motion
  Constant : Constant  Value=M
  D : Gain  Orientation=left  Gain=D  Multiplication=Matrix(K*u)
  G : Gain  Orientation=left  Gain=G  Multiplication=Matrix(K*u)
  Sum : Sum  Inputs=+--
  eta : Outport  InitialOutput=0
  nu : Outport  Port=2  InitialOutput=0
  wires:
  tau/1 -> Sum/1
  Sum/1 -> 6 DOF Eqs. of motion/2
  D/1 -> Sum/3
  G/1 -> Sum/2
  6 DOF Eqs. of motion/2 -> D/1, nu/1
  6 DOF Eqs. of motion/1 -> G/1, eta/1
  Constant/1 -> 6 DOF Eqs. of motion/1

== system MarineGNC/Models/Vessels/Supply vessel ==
  tau : Inport
  D : Gain  Orientation=left  Gain=D  Multiplication=Matrix(K*u)
  Integrator : Integrator
  Integrator1 : Integrator
  Minv : Gain  Gain=Minv  Multiplication=Matrix(K*u)
  "Rotataion matrix in yaw " : MarineGNC/Library blocks/Axes transformations/Rotataion matrix in yaw 
  Sum : Sum  Inputs=+-
  yaw angle : Fcn  Orientation=left  Expr=u(3)
  eta : Outport  InitialOutput=0
  nu : Outport  Port=2  InitialOutput=0
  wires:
  D/1 -> Sum/2
  Sum/1 -> Minv/1
  Minv/1 -> Integrator/1
  tau/1 -> Sum/1
  "Rotataion matrix in yaw "/1 -> Integrator1/1
  yaw angle/1 -> "Rotataion matrix in yaw "/1  "psi"
  Integrator/1 -> D/1, nu/1, "Rotataion matrix in yaw "/2  "nu"
  Integrator1/1 -> yaw angle/1, eta/1  "eta"

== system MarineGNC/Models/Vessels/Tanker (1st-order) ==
  rudder command : Inport
  Ship model : Subsystem
  Steering machine : MarineGNC/Models/Actuators/Steering machine
  heading angle : Outport
  heading rate : Outport  Port=2
  rudder angle : Outport  Port=3
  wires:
  Steering machine/1 -> rudder angle/1, Ship model/1(rudder angle)
  rudder command/1 -> Steering machine/1
  Ship model/1(heading angle) -> heading angle/1
  Ship model/2(heading rate) -> heading rate/1

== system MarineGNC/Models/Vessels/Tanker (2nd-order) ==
  rudder command : Inport
  Ship model : Subsystem
  Steering machine : MarineGNC/Models/Actuators/Steering machine
  heading angle : Outport
  heading rate : Outport  Port=2
  rudder angle : Outport  Port=3
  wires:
  Ship model/2(heading rate) -> heading rate/1
  Ship model/1(heading angle) -> heading angle/1
  rudder command/1 -> Steering machine/1
  Steering machine/1 -> rudder angle/1, Ship model/1(rudder angle)

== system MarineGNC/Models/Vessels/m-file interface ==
  u : Inport
  xo : Inport  Port=2
  Integrator : Integrator  InitialConditionSource=external  InitialCondition=[1 1]  UpperSaturationLimit=10  LowerSaturationLimit=-10
  Mux1 : Mux  Inputs=2
  m-file : MATLABFcn  MATLABFcn=feval(vessmodel,u(1:dimx_model),u(dimx_model+1:length(u)))  Output1D=off
  x : Outport
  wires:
  m-file/1 -> Integrator/1
  Integrator/1 -> Mux1/1, x/1
  Mux1/1 -> m-file/1
  u/1 -> Mux1/2
  xo/1 -> Integrator/2

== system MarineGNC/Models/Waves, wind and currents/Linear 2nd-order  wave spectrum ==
  white noise : Inport
  Linear 2nd-order wave spectrum : TransferFcn  Numerator=[0.5 0]  Denominator=[1 2*0.1*1.2 1.2^2]
  wave amplitude : Outport
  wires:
  Linear 2nd-order wave spectrum/1 -> wave amplitude/1
  white noise/1 -> Linear 2nd-order wave spectrum/1

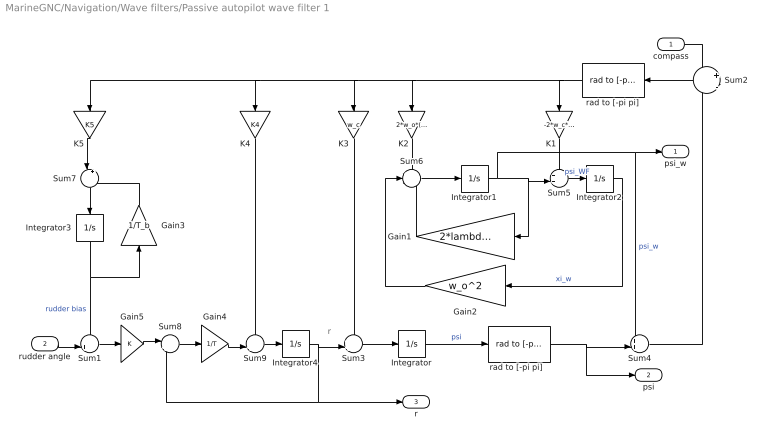
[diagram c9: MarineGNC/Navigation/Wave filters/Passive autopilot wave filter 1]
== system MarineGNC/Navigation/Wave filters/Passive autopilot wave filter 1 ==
  note: r
  compass : Inport
  rudder angle : Inport  Port=2
  Gain1 : Gain  Orientation=left  Gain=2*lambda*w_o
  Gain2 : Gain  Orientation=left  Gain=w_o^2
  Gain3 : Gain  Orientation=up  Gain=1/T_b
  Gain4 : Gain  Gain=1/T
  Gain5 : Gain  Gain=K
  Integrator{,1..2,4} (4 alike) : Integrator
  Integrator3 : Integrator  Orientation=down
  K1 : Gain  Orientation=down  Gain=-2*w_c*(1.0-lambda)/w_o
  K2 : Gain  Orientation=down  Gain=2*w_o*(1.0-lambda)
  K3 : Gain  Orientation=down  Gain=w_c
  K4 : Gain  Orientation=down  Gain=K4
  K5 : Gain  Orientation=down  Gain=K5
  Sum1 : Sum  Inputs=-+|
  Sum2 : Sum  Orientation=left  Inputs=+|-
  Sum{3..5,9} (4 alike) : Sum  Inputs=++|
  Sum6 : Sum  Inputs=+--
  Sum7 : Sum  Orientation=down  Inputs=|+-
  Sum8 : Sum  Inputs=|+-
  rad to [-pi pi] : MarineGNC/Library blocks/Angle conversion/rad to [-pi pi]  Orientation=left  SimViewingDevice=off  DataTypeOverride=UseLocalSettings  MinMaxOverflowLogging=UseLocalSettings
  "rad to [-pi pi]  " : MarineGNC/Library blocks/Angle conversion/rad to [-pi pi]  SimViewingDevice=off  DataTypeOverride=UseLocalSettings  MinMaxOverflowLogging=UseLocalSettings
  psi_w : Outport
  psi : Outport  Port=2
  r : Outport  Port=3
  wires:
  Sum3/1 -> Integrator/1
  Sum2/1 -> rad to [-pi pi]/1
  rad to [-pi pi]/1 -> K1/1, K2/1, K3/1, K4/1, K5/1
  Integrator/1 -> "rad to [-pi pi]  "/1  "psi"
  "rad to [-pi pi]  "/1 -> Sum4/2, psi/1
  Sum4/1 -> Sum2/2
  K3/1 -> Sum3/1
  Sum6/1 -> Integrator1/1
  Gain1/1 -> Sum6/3
  Gain2/1 -> Sum6/2
  Integrator2/1 -> Gain2/1  "xi_w"
  K1/1 -> Sum5/1
  K2/1 -> Sum6/1
  Sum5/1 -> Integrator2/1  "psi_WF"
  Integrator1/1 -> Sum5/2, Gain1/1, Sum4/1, psi_w/1  "psi_w"
  Sum1/1 -> Gain5/1
  compass/1 -> Sum2/1
  rudder angle/1 -> Sum1/2
  Sum8/1 -> Gain4/1
  Integrator4/1 -> Sum8/2, r/1, Sum3/2
  K5/1 -> Sum7/1
  Sum7/1 -> Integrator3/1
  Integrator3/1 -> Sum1/1, Gain3/1  "rudder bias"
  Gain3/1 -> Sum7/2
  Gain5/1 -> Sum8/1
  Gain4/1 -> Sum9/2
  Sum9/1 -> Integrator4/1
  K4/1 -> Sum9/1

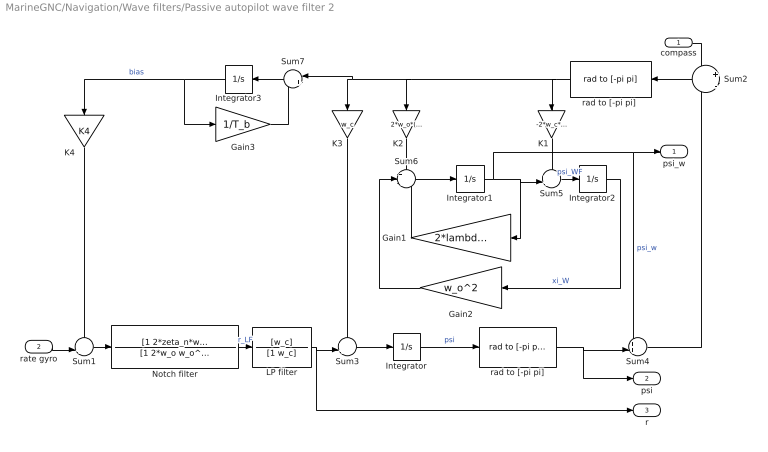
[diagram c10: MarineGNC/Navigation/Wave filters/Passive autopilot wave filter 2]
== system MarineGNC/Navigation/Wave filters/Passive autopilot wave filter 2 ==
  compass : Inport
  rate gyro : Inport  Port=2
  Gain1 : Gain  Orientation=left  Gain=2*lambda*w_o
  Gain2 : Gain  Orientation=left  Gain=w_o^2
  Gain3 : Gain  Gain=1/T_b
  Integrator : Integrator
  Integrator1 : Integrator
  Integrator2 : Integrator
  Integrator3 : Integrator  Orientation=left
  K1 : Gain  Orientation=down  Gain=-2*w_c*(1.0-lambda)/w_o
  K2 : Gain  Orientation=down  Gain=2*w_o*(1.0-lambda)
  K3 : Gain  Orientation=down  Gain=w_c
  K4 : Gain  Orientation=down  Gain=K4
  LP filter : TransferFcn  Numerator=[w_c]  Denominator=[1 w_c]
  Notch filter : TransferFcn  Numerator=[1 2*zeta_n*w_o w_o*w_o]  Denominator=[1 2*w_o w_o^2]
  Sum{1,3..5} (4 alike) : Sum  Inputs=++|
  Sum2 : Sum  Orientation=left  Inputs=+|-
  Sum6 : Sum  Inputs=+--
  Sum7 : Sum  Orientation=left  Inputs=|+-
  rad to [-pi pi] : MarineGNC/Library blocks/Angle conversion/rad to [-pi pi]  SimViewingDevice=off  DataTypeOverride=UseLocalSettings  MinMaxOverflowLogging=UseLocalSettings
  "rad to [-pi pi] " : MarineGNC/Library blocks/Angle conversion/rad to [-pi pi]  Orientation=left  SimViewingDevice=off  DataTypeOverride=UseLocalSettings  MinMaxOverflowLogging=UseLocalSettings
  psi_w : Outport
  psi : Outport  Port=2
  r : Outport  Port=3
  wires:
  K4/1 -> Sum1/1
  Sum3/1 -> Integrator/1
  Sum2/1 -> "rad to [-pi pi] "/1
  "rad to [-pi pi] "/1 -> K1/1, K2/1, K3/1, Sum7/1
  Integrator/1 -> rad to [-pi pi]/1  "psi"
  rad to [-pi pi]/1 -> Sum4/2, psi/1
  Sum4/1 -> Sum2/2
  K3/1 -> Sum3/1
  Sum6/1 -> Integrator1/1
  Gain1/1 -> Sum6/3
  Gain2/1 -> Sum6/2
  Integrator2/1 -> Gain2/1  "xi_W"
  K1/1 -> Sum5/1
  K2/1 -> Sum6/1
  Sum5/1 -> Integrator2/1  "psi_WF"
  Integrator1/1 -> Sum5/2, Gain1/1, Sum4/1, psi_w/1  "psi_w"
  Integrator3/1 -> Gain3/1, K4/1  "bias"
  Notch filter/1 -> LP filter/1  "r_LF"
  Sum1/1 -> Notch filter/1
  LP filter/1 -> Sum3/2, r/1
  Sum7/1 -> Integrator3/1
  Gain3/1 -> Sum7/2
  compass/1 -> Sum2/1
  rate gyro/1 -> Sum1/2

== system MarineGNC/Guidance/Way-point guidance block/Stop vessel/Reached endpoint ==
  IfAction : ActionPort
  Constant : Constant  Value=0
  Stop Simulation : Stop
  stop : Constant  Value=stop
  zero : Outport
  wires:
  Constant/1 -> zero/1
  stop/1 -> Stop Simulation/1

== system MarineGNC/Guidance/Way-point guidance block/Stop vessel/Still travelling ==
  IfAction : ActionPort
  Constant : Constant
  one : Outport
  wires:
  Constant/1 -> one/1

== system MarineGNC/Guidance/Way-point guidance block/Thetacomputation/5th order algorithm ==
  theta : Inport
  IfAction : ActionPort
  Constant1 : Constant
  Constant2 : Constant
  Math Function : Math  Operator=mod
  Mux1 : Mux  Inputs=6
  Product{,1..3} (4 alike) : Product
  theta_vector : Outport
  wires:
  Constant1/1 -> Math Function/2
  Math Function/1 -> Product/1, Product1/2, Product2/2, Product3/2, Mux1/5, Product/2
  theta/1 -> Math Function/1
  Product/1 -> Product1/1, Mux1/4  "t^2"
  Product1/1 -> Product2/1, Mux1/3  "t^3"
  Product2/1 -> Mux1/2, Product3/1  "t^4"
  Product3/1 -> Mux1/1
  Constant2/1 -> Mux1/6
  Mux1/1 -> theta_vector/1

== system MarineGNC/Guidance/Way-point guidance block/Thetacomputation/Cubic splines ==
  theta : Inport
  IfAction : ActionPort
  Constant1 : Constant
  Constant2 : Constant  Value=0
  Mux1 : Mux  Inputs=6
  Product : Product
  Product1 : Product
  theta_vector : Outport
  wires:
  theta/1 -> Product/1, Product/2, Product1/2, Mux1/3
  Product/1 -> Product1/1, Mux1/2  "t^2"
  Mux1/1 -> theta_vector/1
  Product1/1 -> Mux1/1  "t^3"
  Constant1/1 -> Mux1/4
  Constant2/1 -> Mux1/5, Mux1/6

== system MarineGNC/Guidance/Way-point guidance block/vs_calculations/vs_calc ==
  ud : Inport
  xd_theta : Inport  Port=2
  yd_theta : Inport  Port=3
  Math Function : Math  Operator=square
  Math Function1 : Math  Operator=square
  Math Function2 : Math  Operator=sqrt
  Product : Product  Inputs=*/
  Sum : Sum  Inputs=|++
  vs : Outport
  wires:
  Math Function/1 -> Sum/1
  Math Function1/1 -> Sum/2
  Sum/1 -> Math Function2/1
  Math Function2/1 -> Product/2
  xd_theta/1 -> Math Function/1
  ud/1 -> Product/1
  Product/1 -> vs/1  "vs"
  yd_theta/1 -> Math Function1/1

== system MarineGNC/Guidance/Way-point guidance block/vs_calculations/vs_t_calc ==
  xd_theta : Inport
  yd_theta : Inport  Port=2
  ud_dot : Inport  Port=3
  Math Function3 : Math  Operator=square
  Math Function4 : Math  Operator=square
  Math Function5 : Math  Operator=sqrt
  Product7 : Product  Inputs=*/
  Sum3 : Sum  Inputs=|++
  vs_t : Outport
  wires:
  xd_theta/1 -> Math Function3/1
  yd_theta/1 -> Math Function4/1
  Math Function3/1 -> Sum3/1
  Math Function4/1 -> Sum3/2
  Sum3/1 -> Math Function5/1
  Math Function5/1 -> Product7/2
  ud_dot/1 -> Product7/1
  Product7/1 -> vs_t/1

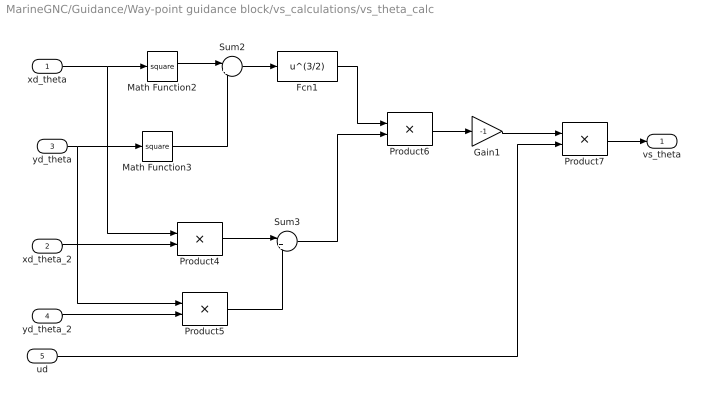
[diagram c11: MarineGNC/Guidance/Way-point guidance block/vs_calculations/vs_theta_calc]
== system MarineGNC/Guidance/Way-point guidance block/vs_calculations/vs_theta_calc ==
  xd_theta : Inport
  xd_theta_2 : Inport  Port=2
  yd_theta : Inport  Port=3
  yd_theta_2 : Inport  Port=4
  ud : Inport  Port=5
  Fcn1 : Fcn  Expr=u^(3/2)
  Gain1 : Gain  Gain=-1
  Math Function2 : Math  Operator=square
  Math Function3 : Math  Operator=square
  Product4 : Product
  Product5 : Product
  Product6 : Product  Inputs=/*
  Product7 : Product
  Sum2 : Sum  Inputs=|++
  Sum3 : Sum  Inputs=|++
  vs_theta : Outport
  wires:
  xd_theta/1 -> Math Function2/1, Product4/1
  yd_theta/1 -> Math Function3/1, Product5/1
  Math Function2/1 -> Sum2/1
  Math Function3/1 -> Sum2/2
  Sum2/1 -> Fcn1/1
  xd_theta_2/1 -> Product4/2
  yd_theta_2/1 -> Product5/2
  Product4/1 -> Sum3/1
  Product5/1 -> Sum3/2
  Fcn1/1 -> Product6/1
  Sum3/1 -> Product6/2
  Product6/1 -> Gain1/1
  Gain1/1 -> Product7/1
  ud/1 -> Product7/2
  Product7/1 -> vs_theta/1

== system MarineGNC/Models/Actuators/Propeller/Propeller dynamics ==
  RPM_c : Inport
  Integrator : Integrator
  Sum : Sum  Inputs=|+-
  rudder angle saturation : Saturate  UpperLimit=delta_max  LowerLimit=-delta_max
  rudder rate saturation : Saturate  UpperLimit=rate_max  LowerLimit=-rate_max
  RPM : Outport
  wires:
  RPM_c/1 -> rudder angle saturation/1
  Integrator/1 -> Sum/2, RPM/1
  rudder angle saturation/1 -> Sum/1
  Sum/1 -> rudder rate saturation/1
  rudder rate saturation/1 -> Integrator/1

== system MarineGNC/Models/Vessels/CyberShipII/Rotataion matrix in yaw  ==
  psi : Inport
  nu : Inport  Port=2
  Fcn : Fcn  Expr=cos(u(1))*u(2)-sin(u(1))*u(3)
  Fcn1 : Fcn  Expr=sin(u(1))*u(2)+cos(u(1))*u(3)
  Fcn2 : Fcn  Expr=u(4)
  Mux : Mux  Inputs=2
  Mux1 : Mux  Inputs=3
  R*nu : Outport
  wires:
  nu/1 -> Mux/2
  psi/1 -> Mux/1
  Mux1/1 -> R*nu/1  "eta_dot"
  Fcn2/1 -> Mux1/3  "psi_dot"
  Fcn1/1 -> Mux1/2  "y_dot"
  Fcn/1 -> Mux1/1  "x_dot"
  Mux/1 -> Fcn/1, Fcn1/1, Fcn2/1

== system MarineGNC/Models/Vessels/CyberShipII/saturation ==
  tau : Inport
  Demux : Demux  Outputs=3
  Mux1 : Mux  Inputs=3
  Saturation : Saturate  UpperLimit=2  LowerLimit=-2
  Saturation1 : Saturate  UpperLimit=1.5  LowerLimit=-1.5
  Saturation2 : Saturate  UpperLimit=1.5  LowerLimit=-1.5
  sat_tau : Outport
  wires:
  Saturation2/1 -> Mux1/3
  Saturation1/1 -> Mux1/2
  Saturation/1 -> Mux1/1
  Demux/3 -> Saturation2/1
  Demux/2 -> Saturation1/1
  Demux/1 -> Saturation/1
  tau/1 -> Demux/1
  Mux1/1 -> sat_tau/1

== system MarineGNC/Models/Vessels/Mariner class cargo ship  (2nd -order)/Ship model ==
  note: heading angle
  rudder angle : Inport
  Integrator : Integrator
  Nomoto 2nd-order model : TransferFcn  Numerator=[K*T3 K]  Denominator=[T1*T2 (T1+T2) 1]
  heading angle : Outport
  heading rate : Outport  Port=2
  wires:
  Integrator/1 -> heading angle/1
  Nomoto 2nd-order model/1 -> Integrator/1, heading rate/1  "heading rate"
  rudder angle/1 -> Nomoto 2nd-order model/1
